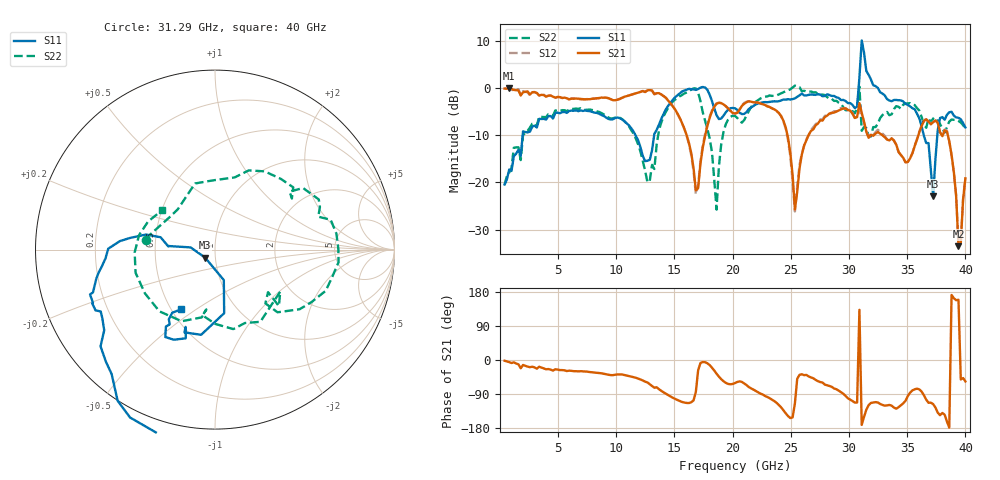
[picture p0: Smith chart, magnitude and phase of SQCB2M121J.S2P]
! Network Analyzer HP8722ES.07.66: Jul 25, 2000 Serial No. US39175408
! 27 Oct 2004  13:09:16
! Frequency  S11  S21  S12  S22
# HZ  S  DB R  50
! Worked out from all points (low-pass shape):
!   201 points, 400 MHz to 40 GHz, reference 50 ohm
!   highest |S21| = -0.10 dB at 796 MHz (marker M1); lowest = -33.5 dB at 39.41 GHz (marker M2)
!   |S21| within 3 dB of the highest: start of sweep to 14.6 GHz; 21.14 GHz to 22.16 GHz (1.023 GHz wide, 4.72 % of centre)
!   lowest |S11| = -23.0 dB at 37.23 GHz (marker M3), VSWR 1.15, Z = 44.6 - j3.99 ohm
!   |S11| at or under -10 dB: start of sweep to 1.954 GHz; 11.64 GHz to 13.25 GHz (1.609 GHz wide, 12.9 % of centre); 36.42 GHz to 37.59 GHz (1.168 GHz wide, 3.16 % of centre)
!   |S22| runs from -25.8 to 0.5 dB; largest |S21 - S12| = 0.12
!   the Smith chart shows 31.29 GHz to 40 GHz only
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4e8  -20.46 -97.0  -0.12 -2.0  -0.07 -1.4  -20.50 -95.2
7.96e8  -17.27 -85.5  -0.10 -5.5  -0.24 -4.9  -17.91 -99.2
7.132e9  -4.87 -102.0  -2.36 -29.9  -2.45 -30.6  -4.54 -132.6
1.2676e10  -15.43 -37.8  -0.49 -59.3  -0.43 -60.1  -19.98 111.2
1.3666e10  -7.77 7.1  -1.09 -77.2  -1.09 -77.7  -8.97 7.7
1.6834e10  -0.40 -11.8  -21.67 -84.4  -22.54 -80.2  -0.09 -92.8
1.8616e10  -5.75 -27.8  -3.35 -36.2  -3.23 -37.1  -25.78 93.2
2.02e10  -4.30 -0.4  -5.41 -60.8  -5.37 -61.4  -5.94 -21.8
2.3368e10  -2.87 -18.1  -4.31 -104.3  -4.31 -105.3  -1.68 -18.4
2.4556e10  -2.47 -96.7  -8.35 -140.6  -8.60 -141.6  -0.67 -21.1
2.5348e10  -2.19 -171.3  -25.75 -114.6  -26.18 -102.2  0.51 -32.5
2.6932e10  -1.43 123.2  -8.75 -48.2  -8.27 -51.4  -0.94 -47.7
3.0694e10  -3.92 20.5  -6.17 -112.3  -6.09 -113.8  -4.19 -115.0
3.0892e10  2.23 1.5  -3.21 132.4  -4.87 129.5  0.29 27.3
3.109e10  10.08 -43.1  -5.23 -171.3  -5.44 -171.1  -9.06 136.9
3.1288e10  7.51 -69.1  -7.14 -150.1  -7.30 -150.0  -8.27 172.1
3.1684e10  2.81 -92.4  -10.56 -119.1  -10.31 -119.8  -10.17 144.0
3.3466e10  -2.67 -148.6  -11.10 -118.6  -10.97 -119.3  -5.78 33.6
3.7228e10  -22.99 -141.0  -7.23 -116.3  -7.19 -116.9  -6.47 -57.9
3.8614e10  -5.16 -114.5  -11.24 -178.4  -11.34 -179.9  -7.13 -114.9
3.9406e10  -6.32 -121.6  -33.53 159.0  -33.25 160.7  -6.98 -178.0
4e10  -8.36 -119.5  -19.15 -56.5  -18.99 -57.0  -8.70 143.5
